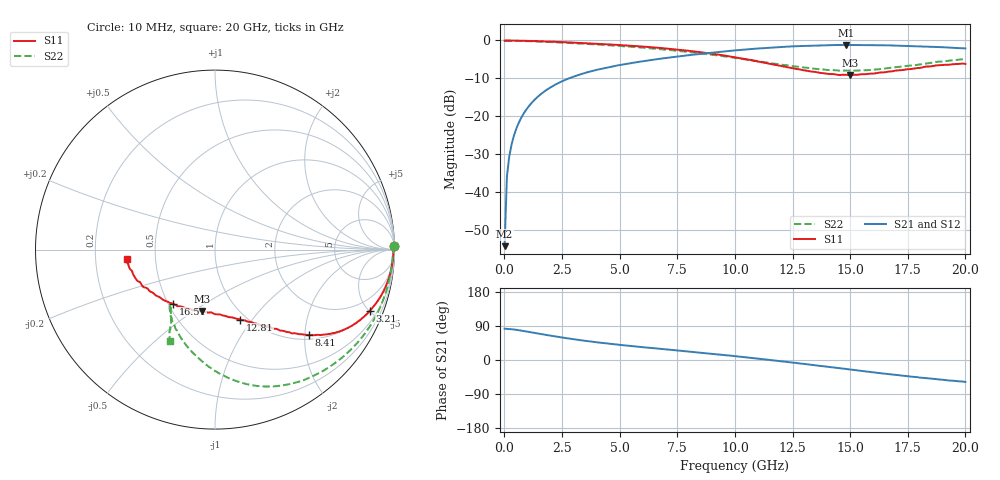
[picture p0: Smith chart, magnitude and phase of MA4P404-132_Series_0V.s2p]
! AWR Design Environment (9226) Thu Aug 19 02:24:33 2021
! Document = '0V'
! nPorts: 2, nXvals: 201
# GHz S DB R 50
!Freq DBS11 AngS11 DBS21 AngS21 DBS12 AngS12 DBS22 AngS22
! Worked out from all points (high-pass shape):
!   201 points, 10 MHz to 20 GHz, reference 50 ohm
!   highest |S21| = -1.20 dB at 14.81 GHz (marker M1); lowest = -54.1 dB at 10 MHz (marker M2)
!   |S21| within 3 dB of the highest: 7.578 GHz to end of sweep
!   lowest |S11| = -9.1 dB at 15.01 GHz (marker M3), VSWR 2.08, Z = 34.5 - j26.9 ohm
!   |S11| at or under -10 dB: nowhere
!   |S22| runs from -8.0 to 0.0 dB; largest |S21 - S12| = 0.035
!   S11 on the Smith chart (normalised r, x): 10 MHz: 19, +86; 3.21 GHz: 1.03, -5.06; 8.41 GHz: 1.10, -2.09; 12.81 GHz: 0.93, -0.88; 16.51 GHz: 0.53, -0.37; 20 GHz: 0.34, -0.05
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0.01  -0.04 1.3  -54.14 82.7  -55.89 70.7  -0.02 1.1
0.11  -0.06 -1.0  -35.82 82.0  -35.83 81.8  -0.08 -1.9
0.21  -0.06 -1.8  -30.59 81.7  -30.61 81.9  -0.09 -3.6
0.31  -0.06 -2.5  -27.45 81.3  -27.44 81.4  -0.10 -5.3
0.61  -0.08 -4.8  -21.86 78.8  -21.87 78.8  -0.13 -10.2
1.01  -0.13 -7.8  -17.73 74.7  -17.73 74.8  -0.19 -16.7
1.61  -0.23 -12.0  -14.01 68.3  -14.01 68.6  -0.32 -25.9
2.31  -0.40 -16.5  -11.33 61.2  -11.33 61.6  -0.52 -35.7
3.21  -0.65 -21.5  -9.11 53.1  -9.10 53.6  -0.82 -46.6
3.41  -0.71 -22.6  -8.73 51.4  -8.72 52.0  -0.88 -48.8
4.91  -1.20 -29.2  -6.59 40.6  -6.58 41.4  -1.43 -63.0
6.71  -1.96 -36.0  -4.87 29.9  -4.83 30.9  -2.27 -76.7
8.41  -3.03 -42.4  -3.62 20.1  -3.57 21.2  -3.34 -89.2
10.01  -4.43 -49.4  -2.63 10.1  -2.56 11.5  -4.60 -101.9
12.81  -7.64 -70.2  -1.50 -9.1  -1.45 -7.8  -6.99 -123.4
13.41  -8.26 -77.2  -1.37 -13.3  -1.32 -12.1  -7.42 -126.1
14.81  -9.05 -98.1  -1.20 -23.6  -1.19 -22.2  -7.93 -128.3
15.01  -9.12 -102.2  -1.21 -25.2  -1.19 -23.8  -7.94 -128.6
16.51  -8.38 -127.8  -1.28 -36.2  -1.29 -34.0  -7.39 -125.2
16.71  -8.19 -130.3  -1.32 -37.6  -1.30 -35.5  -7.26 -124.4
18.71  -6.60 -158.3  -1.74 -50.2  -1.73 -48.9  -5.70 -119.1
20  -6.18 -173.7  -2.10 -57.9  -2.13 -56.3  -4.88 -116.3
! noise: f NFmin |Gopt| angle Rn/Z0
0.01  0  1  0  2e-20
2.21  0  1  0  2e-20
4.41  0  1  0  2e-20
6.61  0  1  0  2e-20
8.81  0  1  0  2e-20
11.11  0  1  0  2e-20
13.31  0  1  0  2e-20
15.51  0  1  0  2e-20
17.71  0  1  0  2e-20
20  0  1  0  2e-20
